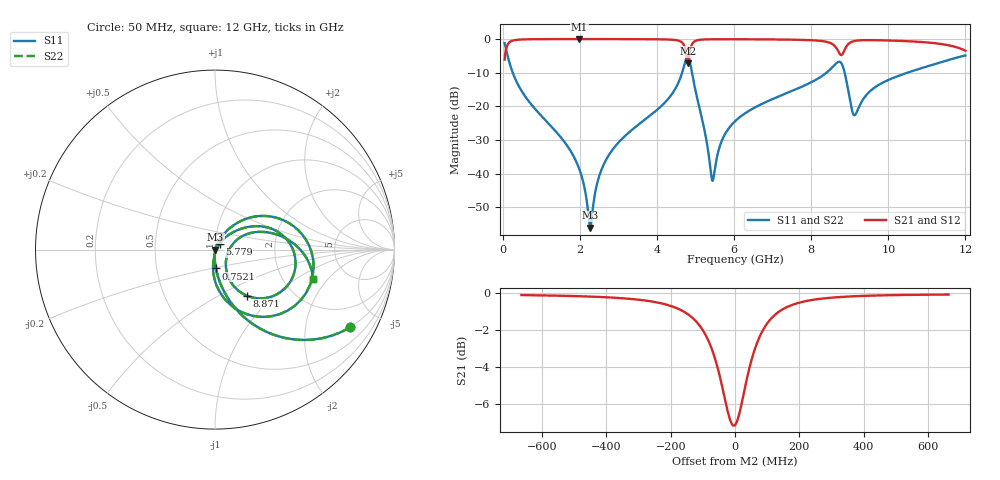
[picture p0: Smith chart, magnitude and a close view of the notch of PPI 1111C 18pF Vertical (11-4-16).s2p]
# GHz S MA R 50
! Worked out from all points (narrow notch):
!   1601 points, 50 MHz to 12 GHz, reference 50 ohm
!   highest |S21| = -0.01 dB at 1.992 GHz (marker M1); lowest = -7.2 dB at 4.808 GHz (marker M2)
!   notch at M2: 7.0 dB deep, 111 MHz wide at half that depth
!   lowest |S11| = -56.1 dB at 2.268 GHz (marker M3), VSWR 1.00, Z = 50.2 - j0.0445 ohm
!   |S11| at or under -10 dB: 260.3 MHz to 4.654 GHz (4.394 GHz wide, 179 % of centre); 4.909 GHz to 8.398 GHz (3.49 GHz wide, 52.4 % of centre); 8.868 GHz to 10.5 GHz (1.63 GHz wide, 16.8 % of centre)
!   |S22| runs from -56.1 to -1.2 dB; largest |S21 - S12| = 0
!   S11 on the Smith chart (normalised r, x): 50 MHz: 0.98, -3.48; 752.1 MHz: 0.99, -0.21; 5.779 GHz: 1.05, +0.06; 8.871 GHz: 1.22, -0.69; 12 GHz: 2.89, -1.41
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0.05  0.8688 -29.9  0.4949 60.1  0.4949 60.1  0.8688 -29.9
0.2441875  0.3352 -71.6  0.9416 18.3  0.9416 18.3  0.3352 -71.6
0.7520625  0.1049 -87.4  0.9935 2.1  0.9935 2.1  0.1049 -87.4
1.991875  0.01146 -92.4  0.9984 -9.7  0.9984 -9.7  0.01146 -92.4
2.044156  0.009291 -91.0  0.9984 -10.1  0.9984 -10.1  0.009291 -91.0
2.268219  0.00157 -16.4  0.9983 -11.7  0.9983 -11.7  0.00157 -16.4
2.484812  0.008472 65.3  0.9981 -13.3  0.9981 -13.3  0.008472 65.3
2.73875  0.01826 69.1  0.9979 -15.2  0.9979 -15.2  0.01826 69.1
4.038312  0.09219 61.2  0.9911 -26.0  0.9911 -26.0  0.09219 61.2
4.665687  0.3326 34.3  0.8714 -42.8  0.8714 -42.8  0.3326 34.3
4.807594  0.5622 -25.4  0.4377 -23.5  0.4377 -23.5  0.5622 -25.4
4.874812  0.4039 -63.3  0.7282 -4.7  0.7282 -4.7  0.4039 -63.3
4.971906  0.205 -86.9  0.9199 -14.1  0.9199 -14.1  0.205 -86.9
5.4275  0.008125 -38.6  0.9917 -27.5  0.9917 -27.5  0.008125 -38.6
5.778531  0.03974 50.8  0.9936 -31.5  0.9936 -31.5  0.03974 50.8
6.025  0.05984 51.6  0.9932 -33.9  0.9932 -33.9  0.05984 51.6
8.019156  0.2303 33.6  0.9594 -53.1  0.9594 -53.1  0.2303 33.6
8.691344  0.4529 -8.1  0.6783 -65.2  0.6783 -65.2  0.4529 -8.1
8.870594  0.3124 -55.3  0.6965 -38.4  0.6965 -38.4  0.3124 -55.3
9.124531  0.07358 -16.8  0.9351 -46.8  0.9351 -46.8  0.07358 -16.8
10.01331  0.248 23.2  0.9515 -62.9  0.9515 -62.9  0.248 23.2
12  0.5699 -16.8  0.6712 -89.8  0.6712 -89.8  0.5699 -16.8
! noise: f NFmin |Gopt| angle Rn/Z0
0.05  0.0003826  0.8713  1.231  0.0006402
1.372  0.00395  0.6878  7.306  0.002449
2.701  0.006807  0.6538  13.89  0.003691
4.031  0.01281  0.7189  20.4  0.008741
5.36  0.02113  0.7712  27.28  0.0178
6.682  0.01678  0.6698  33.09  0.009008
8.012  0.03056  0.7756  39.3  0.02475
9.341  0.05012  0.8399  45.56  0.05645
10.67  0.04506  0.8075  50.86  0.03982
12  0.15  0.933  56.66  0.3859
